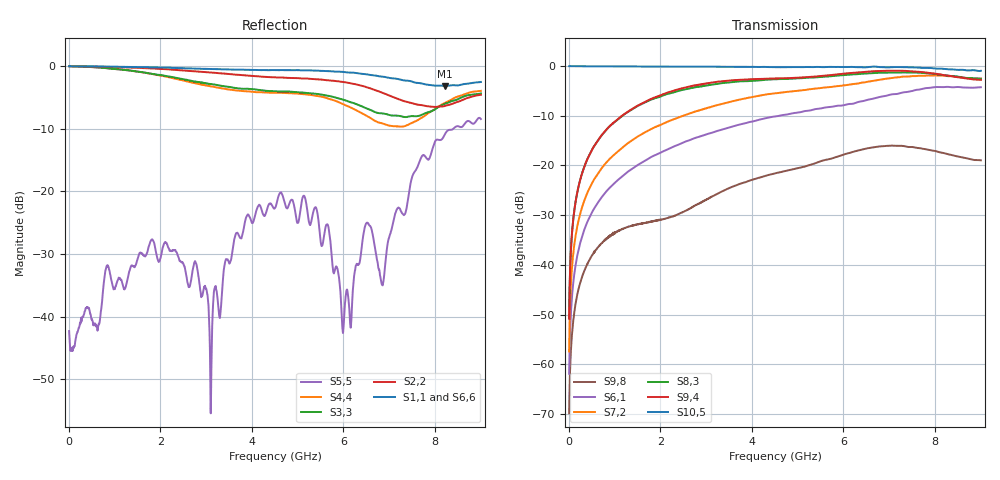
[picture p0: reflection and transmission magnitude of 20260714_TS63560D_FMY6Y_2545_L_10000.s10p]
# GHz S DB R 50
! CMT, SN0916, 25263762, 26.7.0
! Date: 15.07.2026 13:41:22
! Data: Format
! Freq S1.1:dB/Ang S1.2:dB/Ang S1.3:dB/Ang S1.4:dB/Ang S1.5:dB/Ang S1.6:dB/Ang S1.7:dB/Ang S1.8:dB/Ang S1.9:dB/Ang S1.10:dB/Ang
!  S2.1:dB/Ang S2.2:dB/Ang S2.3:dB/Ang S2.4:dB/Ang S2.5:dB/Ang S2.6:dB/Ang S2.7:dB/Ang S2.8:dB/Ang S2.9:dB/Ang S2.10:dB/Ang
!  S3.1:dB/Ang S3.2:dB/Ang S3.3:dB/Ang S3.4:dB/Ang S3.5:dB/Ang S3.6:dB/Ang S3.7:dB/Ang S3.8:dB/Ang S3.9:dB/Ang S3.10:dB/Ang
!  S4.1:dB/Ang S4.2:dB/Ang S4.3:dB/Ang S4.4:dB/Ang S4.5:dB/Ang S4.6:dB/Ang S4.7:dB/Ang S4.8:dB/Ang S4.9:dB/Ang S4.10:dB/Ang
!  S5.1:dB/Ang S5.2:dB/Ang S5.3:dB/Ang S5.4:dB/Ang S5.5:dB/Ang S5.6:dB/Ang S5.7:dB/Ang S5.8:dB/Ang S5.9:dB/Ang S5.10:dB/Ang
!  S6.1:dB/Ang S6.2:dB/Ang S6.3:dB/Ang S6.4:dB/Ang S6.5:dB/Ang S6.6:dB/Ang S6.7:dB/Ang S6.8:dB/Ang S6.9:dB/Ang S6.10:dB/Ang
!  S7.1:dB/Ang S7.2:dB/Ang S7.3:dB/Ang S7.4:dB/Ang S7.5:dB/Ang S7.6:dB/Ang S7.7:dB/Ang S7.8:dB/Ang S7.9:dB/Ang S7.10:dB/Ang
!  S8.1:dB/Ang S8.2:dB/Ang S8.3:dB/Ang S8.4:dB/Ang S8.5:dB/Ang S8.6:dB/Ang S8.7:dB/Ang S8.8:dB/Ang S8.9:dB/Ang S8.10:dB/Ang
!  S9.1:dB/Ang S9.2:dB/Ang S9.3:dB/Ang S9.4:dB/Ang S9.5:dB/Ang S9.6:dB/Ang S9.7:dB/Ang S9.8:dB/Ang S9.9:dB/Ang S9.10:dB/Ang
!  S10.1:dB/Ang S10.2:dB/Ang S10.3:dB/Ang S10.4:dB/Ang S10.5:dB/Ang S10.6:dB/Ang S10.7:dB/Ang S10.8:dB/Ang S10.9:dB/Ang S10.10:dB/Ang
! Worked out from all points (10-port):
!   2001 points, 10 MHz to 9 GHz, reference 50 ohm
!   strongest paths, dB at 10 MHz, 2.257 GHz, 4.505 GHz, 6.753 GHz, 9 GHz:
!     S10,5: -0.1, -0.2, -0.2, -0.2, -1.0
!     S9,4: -50.8, -5.1, -2.5, -1.0, -2.8
!     S8,3: -50.6, -5.4, -2.7, -1.4, -2.6
!     S7,2: -57.4, -10.9, -5.5, -2.8, -2.6
!     S6,1: -61.9, -16.4, -10.2, -6.3, -4.3
!     S9,8: -69.8, -30.3, -21.6, -16.2, -19.0
!   lowest |S11| = -3.2 dB at 8.213 GHz (marker M1), VSWR 5.55, Z = 11.1 - j23.5 ohm
!   |S11| at or under -10 dB: nowhere
